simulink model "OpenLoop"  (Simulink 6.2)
settings: Solver=ode45  StartTime=0.0  StopTime=100  RelTol=1e-3
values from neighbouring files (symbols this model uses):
  Agu = [    [guidance.m]
  Ave = [    [pitch_vehi3.m]    (also in Siso_Anal.m; vehi_latan2.m; vehi_ldes.m)
  Bgu = [    [guidance.m]
  Bve = [    [pitch_vehi3.m]    (also in Siso_Anal.m; vehi_latan2.m; vehi_ldes.m)
  Cgu = [    [guidance.m]
  Cve = [    [pitch_vehi3.m]    (also in Siso_Anal.m; vehi_latan2.m; vehi_ldes.m)
  Dgu = [    [guidance.m]
  Dve = [    [pitch_vehi3.m]    (also in Siso_Anal.m; vehi_latan2.m; vehi_ldes.m)
  x0 = [0.1, -0.08, 0.18, 9000, 50, zeros(1,8)]    [run.m]

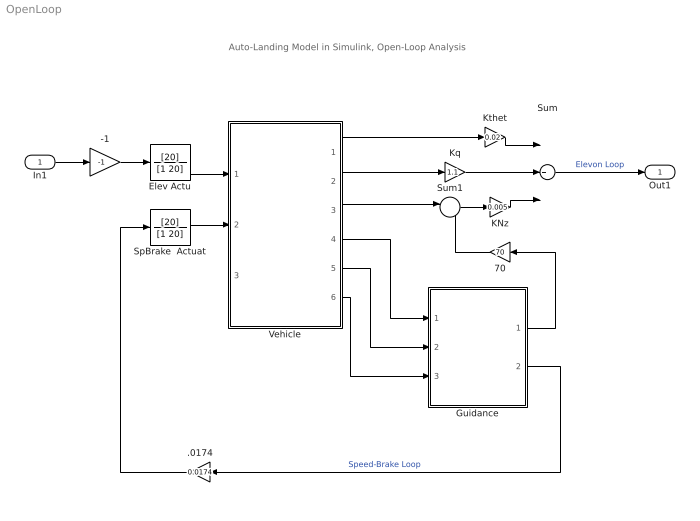
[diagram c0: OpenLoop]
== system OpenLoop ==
  note: Auto-Landing Model in Simulink, Open-Loop Analysis
  In1 : Inport  Port=1  LatchInput=off
  -1 : Gain  Gain=-1
  .0174 : Gain  Orientation=left  Gain=0.0174
  70 : Gain  Orientation=left  Gain=70
  Elev Actu : TransferFcn  Numerator=[20]  Denominator=[1 20]
  Guidance : Subsystem
  KNz : Gain  Gain=0.005
  Kq : Gain  Gain=1.1
  Kthet : Gain  Gain=0.02
  SpBrake  Actuat : TransferFcn  Numerator=[20]  Denominator=[1 20]
  Sum : Sum  Inputs=+++  OutScaling=2^-10
  Sum1 : Sum  Inputs=|-+
  Vehicle : Subsystem
  Out1 : Outport
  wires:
  Elev Actu/1 -> Vehicle/1(Elevon)
  SpBrake  Actuat/1 -> Vehicle/2(Sp_Brake)
  Vehicle/1(theta) -> Kthet/1
  Kthet/1 -> Sum/1
  Vehicle/2(q) -> Kq/1
  Kq/1 -> Sum/2
  KNz/1 -> Sum/3
  Vehicle/3(Acc_Z) -> Sum1/1
  Sum1/1 -> KNz/1
  Vehicle/6(dH) -> Guidance/3(dH)
  Vehicle/5(dH-dot) -> Guidance/2(H-dot)
  Vehicle/4(dV) -> Guidance/1(dV)
  70/1 -> Sum1/2
  .0174/1 -> SpBrake  Actuat/1
  In1/1 -> -1/1
  -1/1 -> Elev Actu/1
  Guidance/1(Nz-com) -> 70/1
  Guidance/2(SpBrak-com) -> .0174/1  "Speed-Brake Loop"
  Sum/1 -> Out1/1  "Elevon Loop"

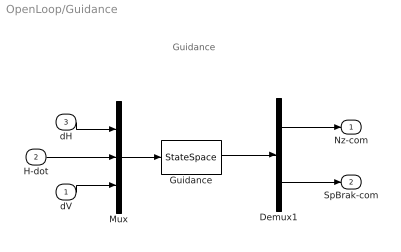
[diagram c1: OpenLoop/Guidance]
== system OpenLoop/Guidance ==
  note: Guidance
  dV : Inport  Port=1  LatchInput=off
  H-dot : Inport  Port=2  LatchInput=off
  dH : Inport  Port=3  LatchInput=off
  Demux1 : Demux  Outputs=2
  Guidance : StateSpace  A=Agu  B=Bgu  C=Cgu  D=Dgu
  Mux : Mux  Inputs=3
  Nz-com : Outport
  SpBrak-com : Outport  Port=2
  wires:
  dH/1 -> Mux/1
  H-dot/1 -> Mux/2
  dV/1 -> Mux/3
  Mux/1 -> Guidance/1
  Guidance/1 -> Demux1/1
  Demux1/2 -> SpBrak-com/1
  Demux1/1 -> Nz-com/1

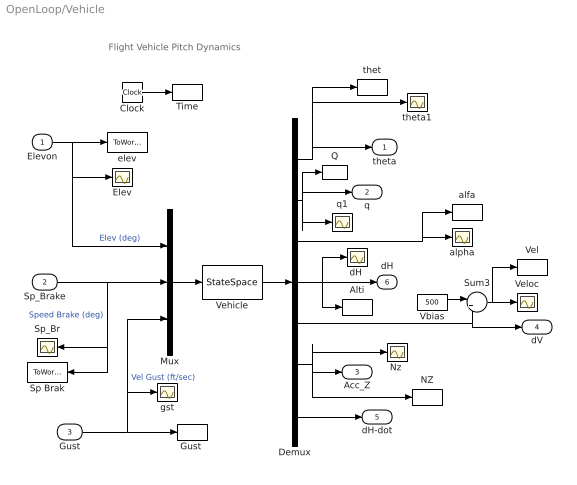
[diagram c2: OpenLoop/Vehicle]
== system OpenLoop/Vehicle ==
  note: Flight Vehicle Pitch Dynamics
  Elevon : Inport  Port=1  LatchInput=off
  Sp_Brake : Inport  Port=2  LatchInput=off
  Gust : Inport  Port=3  LatchInput=off
  Alti : ToWorkspace  VariableName=Alti  SampleTime=-1  SaveFormat=Array
  Clock : Clock
  Demux : Demux  Outputs=7
  Elev : Scope
  "Gust " : ToWorkspace  VariableName=Gust  SampleTime=-1  SaveFormat=Array
  Mux : Mux  Inputs=3
  NZ : ToWorkspace  VariableName=Nz  SampleTime=-1  SaveFormat=Array
  "Nz " : Scope
  Q : ToWorkspace  VariableName=q  SampleTime=-1  SaveFormat=Array
  Sp Brak : ToWorkspace  VariableName=SpBrake  SampleTime=-1  SaveFormat=Array
  Sp_Br : Scope
  Sum3 : Sum  Inputs=|++
  Time : ToWorkspace  VariableName=time  SampleTime=-1  SaveFormat=Array
  Vbias : Constant  Value=500
  Vehicle : StateSpace  A=Ave  B=Bve  C=Cve  D=Dve  X0=x0
  Vel : ToWorkspace  VariableName=Vel  SampleTime=-1  SaveFormat=Array
  Veloc : Scope
  alfa : ToWorkspace  VariableName=alpha  SampleTime=-1  SaveFormat=Array
  alpha : Scope
  "dH " : Scope
  elev : ToWorkspace  VariableName=Elevon  SampleTime=-1  SaveFormat=Array
  gst : Scope
  q1 : Scope
  thet : ToWorkspace  VariableName=theta  SampleTime=-1  SaveFormat=Array
  theta1 : Scope
  theta : Outport
  q : Outport  Port=2
  Acc_Z : Outport  Port=3
  dV : Outport  Port=4
  dH-dot : Outport  Port=5
  dH : Outport  Port=6
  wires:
  Mux/1 -> Vehicle/1
  Vehicle/1 -> Demux/1
  Demux/1 -> theta/1, theta1/1, thet/1
  Demux/2 -> q/1, Q/1, q1/1
  Demux/3 -> alpha/1, alfa/1
  Demux/4 -> dH/1, "dH "/1, Alti/1
  Demux/5 -> dV/1, Sum3/2
  Gust/1 -> "Gust "/1, Mux/3, gst/1  "Vel Gust (ft/sec)"
  Demux/6 -> Acc_Z/1, "Nz "/1, NZ/1
  Demux/7 -> dH-dot/1
  Elevon/1 -> elev/1, Mux/1, Elev/1  "Elev (deg)"
  Sp_Brake/1 -> Mux/2, Sp Brak/1, Sp_Br/1  "Speed Brake (deg)"
  Clock/1 -> Time/1
  Vbias/1 -> Sum3/1
  Sum3/1 -> Veloc/1, Vel/1
